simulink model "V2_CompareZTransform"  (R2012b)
settings: Solver=ode4  SolverMode=SingleTasking  StartTime=0.0  StopTime=5  FixedStep=1e-4  RelTol=1e-3

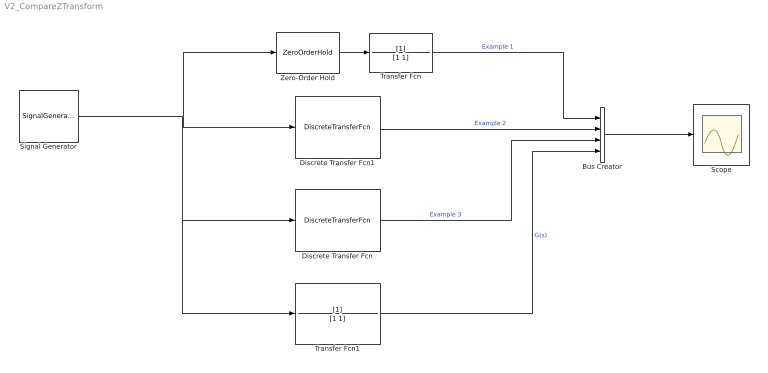
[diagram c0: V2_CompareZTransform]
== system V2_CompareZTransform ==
  Bus Creator : BusCreator  Inputs=4
  Discrete Transfer Fcn : DiscreteTransferFcn  Numerator=[0.1 0]  Denominator=[1 -exp(-0.1)]  SampleTime=0.1
  Discrete Transfer Fcn1 : DiscreteTransferFcn  Numerator=[0.09516]  Denominator=[1 -exp(-0.1)]  SampleTime=0.1
  Scope : Scope
  Signal Generator : SignalGenerator  Amplitude=10
  Transfer Fcn : TransferFcn  Denominator=[1 1]
  Transfer Fcn1 : TransferFcn  Denominator=[1 1]
  Zero-Order Hold : ZeroOrderHold  SampleTime=0.1
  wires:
  Zero-Order Hold/1 -> Transfer Fcn/1
  Transfer Fcn/1 -> Bus Creator/1  "Example 1"
  Signal Generator/1 -> Discrete Transfer Fcn1/1, Zero-Order Hold/1, Discrete Transfer Fcn/1, Transfer Fcn1/1
  Bus Creator/1 -> Scope/1
  Discrete Transfer Fcn/1 -> Bus Creator/3  "Example 3"
  Discrete Transfer Fcn1/1 -> Bus Creator/2  "Example 2"
  Transfer Fcn1/1 -> Bus Creator/4  "G(s)"
